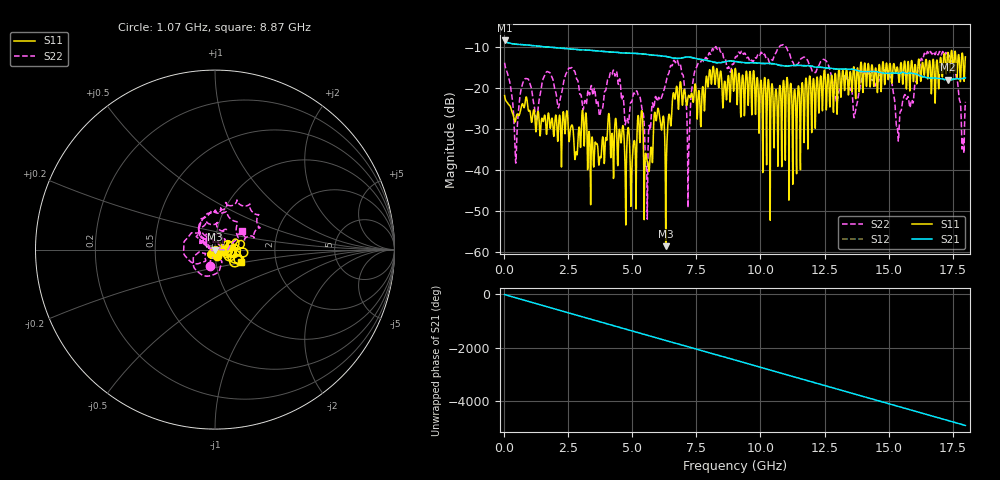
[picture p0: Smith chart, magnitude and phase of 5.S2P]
!Agilent Technologies,E5071C,MY46316741,A.11.02
!Date: Thu Sep 29 15:35:02 2022
!Data & Calibration Information:
!Freq	S11:SOLT2(ON)	S21:SOLT2(ON)	S12:SOLT2(ON)	S22:SOLT2(ON)
!PortZ  Port1:50+j0  Port2:50+j0
!Above PortZ is port z conversion or system Z0 setting when saving the data.
!When reading, reference impedance value at option line is always used.
# Hz S dB R 50
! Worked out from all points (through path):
!   1800 points, 10 MHz to 18 GHz, reference 50 ohm
!   highest |S21| = -8.41 dB at 10 MHz (marker M1); lowest = -18.0 dB at 17.32 GHz (marker M2)
!   group delay of S21, straight-line fit = 757 ps
!   lowest |S11| = -58.6 dB at 6.3 GHz (marker M3), VSWR 1.00, Z = 50 - j0.113 ohm
!   |S11| at or under -10 dB: start of sweep to end of sweep
!   |S22| runs from -52.0 to -9.4 dB; largest |S21 - S12| = 0.016
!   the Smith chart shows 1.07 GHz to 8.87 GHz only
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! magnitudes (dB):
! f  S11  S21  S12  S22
! 10 MHz  -21.8  -8.4  -8.4  -13.8
! 450 MHz  -27.5  -9.3  -9.3  -38.3
! 830 MHz  -22.6  -9.5  -9.5  -17.7
! 1.24 GHz  -30.7  -9.8  -9.8  -28.1
! 3.01 GHz  -28.7  -10.7  -10.7  -22.2
! 4.32 GHz  -28.4  -11.3  -11.3  -17.1
! 4.78 GHz  -34.6  -11.5  -11.5  -27.3
! 5.25 GHz  -27.9  -11.6  -11.6  -22.0
! 5.56 GHz  -37.3  -11.8  -11.8  -40.7
! 6.01 GHz  -25.0  -12.1  -12.1  -22.4
! 6.3 GHz  -58.6  -12.3  -12.3  -19.0
! 6.82 GHz  -22.8  -12.8  -12.8  -14.4
! 7.18 GHz  -22.0  -12.4  -12.5  -42.5
! 7.54 GHz  -26.5  -12.9  -13.0  -14.3
! 9.01 GHz  -15.3  -13.6  -13.6  -12.6
! 12.01 GHz  -27.1  -14.7  -14.7  -15.8
! 13.7 GHz  -20.7  -15.6  -15.6  -25.9
! 15.01 GHz  -16.4  -16.4  -16.4  -16.3
! 15.37 GHz  -15.9  -16.4  -16.4  -32.0
! 16.34 GHz  -13.9  -17.2  -17.3  -13.1
! 17.32 GHz  -11.3  -18.0  -18.0  -12.5
! 18 GHz  -12.4  -17.6  -17.7  -23.4
